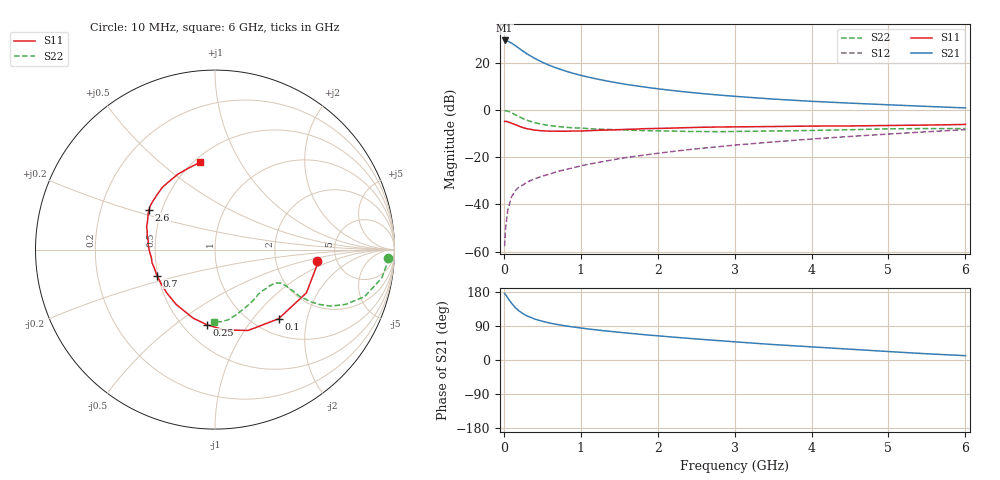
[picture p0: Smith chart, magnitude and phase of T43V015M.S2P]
! Infineon Technologies  Discrete & RF Semiconductors
! BFR182T
! Si NPN RF Bipolar Junction Transistor in SC75
! VCE = 3 V  IC = 15 mA
! Common Emitter S-Parameters:  October  1999
# GHz  S  MA  R  50
!  f  S11  S21  S12  S22
! GHz  MAG  ANG  MAG  ANG  MAG  ANG  MAG  ANG
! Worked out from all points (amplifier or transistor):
!   36 points, 10 MHz to 6 GHz, reference 50 ohm
!   highest |S21| = 29.4 dB at 10 MHz (marker M1)
!   |S21| within 3 dB of that: start of sweep to 183.6 MHz
!   unconditionally stable (mu >= 1): 775.1 MHz to 3.68 GHz
!   at 250 MHz: K = 0.58, MSG = 28.3 dB, |S12| = -31.8 dB
!   at 1.4 GHz: K = 1.10, MAG = 14.7 dB, |S12| = -21.2 dB
!   at 6 GHz: K = 0.84, MSG = 4.6 dB, |S12| = -8.4 dB
!   S11 on the Smith chart (normalised r, x): 10 MHz: 3.53, -0.64; 100 MHz: 1.28, -1.36; 250 MHz: 0.65, -0.66; 700 MHz: 0.49, -0.16; 2.6 GHz: 0.42, +0.23; 6 GHz: 0.54, +0.69
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0.01  0.5703 -6.2  29.65 175.6  0.0013 71.0  0.9624 -2.7
0.02  0.5748 -8.8  29.42 173.5  0.0028 102.4  0.9659 -3.8
0.05  0.5634 -25.3  28.77 163.7  0.0074 83.7  0.9431 -9.6
0.1  0.5234 -47.4  26.05 149.8  0.0144 74.1  0.8734 -17.5
0.15  0.4869 -67.7  22.98 138.0  0.0195 67.0  0.7884 -22.8
0.2  0.4512 -83.4  20.08 129.1  0.0237 64.6  0.7161 -26.1
0.25  0.4207 -96.3  17.55 122.2  0.0258 62.1  0.6534 -27.8
0.3  0.401 -107.7  15.48 116.6  0.0296 62.0  0.6063 -28.6
0.4  0.3742 -125.5  12.4 108.1  0.0346 61.5  0.5358 -28.9
0.5  0.3611 -138.2  10.25 102.2  0.0396 62.9  0.4955 -28.0
0.6  0.355 -147.9  8.701 97.4  0.044 63.9  0.4664 -27.6
0.7  0.3546 -155.9  7.569 93.5  0.0497 65.2  0.4452 -27.1
0.9  0.3585 -168.4  5.979 87.2  0.0593 67.2  0.4178 -26.9
1.1  0.3637 -177.5  4.95 81.8  0.0707 68.4  0.4029 -27.6
1.3  0.3742 175.2  4.231 77.2  0.0814 69.3  0.389 -28.8
1.6  0.3887 166.6  3.464 71.1  0.0985 69.3  0.3747 -31.1
2.2  0.4132 155.0  2.571 60.4  0.1322 69.1  0.3563 -38.0
2.6  0.4299 148.7  2.207 54.0  0.1556 68.2  0.3484 -43.4
3.5  0.4453 136.0  1.699 40.8  0.2098 65.0  0.3583 -56.4
4.5  0.4582 123.4  1.394 28.5  0.2744 60.0  0.3811 -71.9
5.5  0.4779 107.6  1.189 16.4  0.3449 54.0  0.4029 -85.2
6  0.4929 99.9  1.102 11.4  0.3818 50.2  0.4023 -90.5
